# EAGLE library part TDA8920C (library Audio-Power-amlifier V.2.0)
The TDA8920C is a high-efficiency class-D audio power amplifier. The typical output power is 2 ´ 110 W with a speaker load impedance of 4 W. The TDA8920C is available in both HSOP24 and DBS23P power packages. The amplifier operates over a wide supply voltage range from ±12.5 V to ±32.5 V and features low quiescent current consumption.
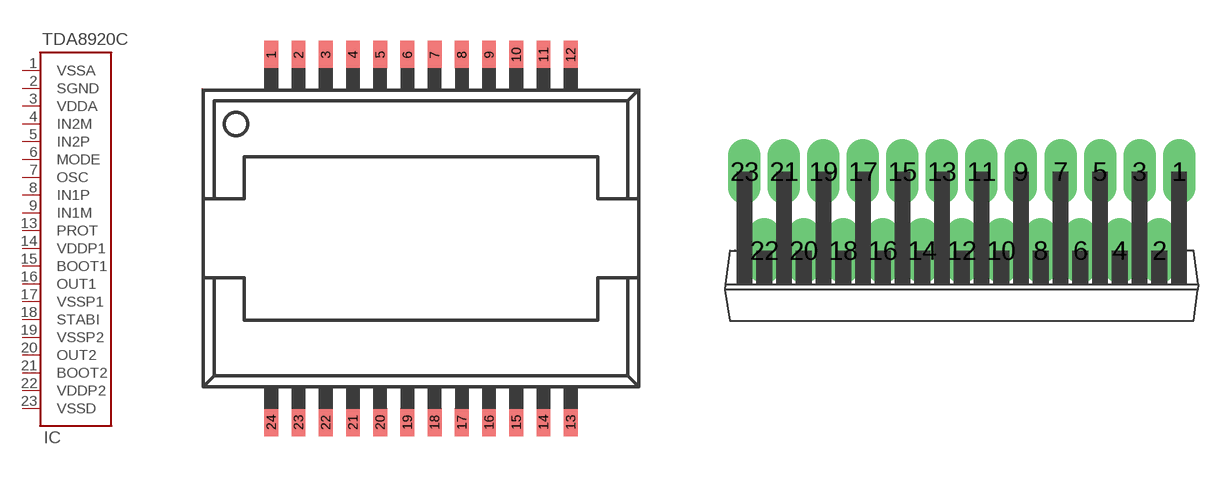
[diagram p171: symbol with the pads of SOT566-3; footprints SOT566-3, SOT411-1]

Designator prefix IC

## TDA8920CTDA8920CTH  [SOT566-3]
1  VSSA  pwr
2  SGND  pwr
3  VDDA  pwr
4  IN2M  in
5  IN2P  in
6  MODE  in
7  OSC  in
8  IN1P  in
9  IN1M  in
13  PROT
14  VDDP1  pwr
15  BOOT1
16  OUT1  out
17  VSSP1  pwr
18  STABI  pwr
19  VSSP2  pwr
20  OUT2
21  BOOT2  out
22  VDDP2  pwr
23  VSSD  pwr

## TDA8920CTDA8920CJ  [SOT411-1]
1  MODE  in
2  IN2P  in
3  IN2M  in
4  VDDA  pwr
5  SGND  pwr
6  VSSA  pwr
7  VSSD  pwr
8  VDDP2  pwr
9  BOOT2  out
10  OUT2
11  VSSP2  pwr
12  STABI  pwr
13  VSSP1  pwr
14  OUT1  out
15  BOOT1
16  VDDP1  pwr
17  PROT
21  IN1M  in
22  IN1P  in
23  OSC  in

## Footprint SOT566-3 (pad centres in mm)
smd 0.508 x 1.016: 1 -5.5,6.75; 2 -4.5,6.75; 3 -3.5,6.75; 4 -2.5,6.75; 5 -1.5,6.75; 6 -0.5,6.75; 7 0.5,6.75; 8 1.5,6.75; 9 2.5,6.75; 10 3.5,6.75; 11 4.5,6.75; 12 5.5,6.75; 13 5.5,-6.75; 14 4.5,-6.75; 15 3.5,-6.75; 16 2.5,-6.75; 17 1.5,-6.75; 18 0.5,-6.75; 19 -0.5,-6.75; 20 -1.5,-6.75; 21 -2.5,-6.75; 22 -3.5,-6.75; 23 -4.5,-6.75; 24 -5.5,-6.75

## Footprint SOT411-1 (pad centres in mm)
drill 1.4 long: 1 13.97,5.08; 2 12.7,0; 3 11.43,5.08; 4 10.16,0; 5 8.89,5.08; 6 7.62,0; 7 6.35,5.08; 8 5.08,0; 9 3.81,5.08; 10 2.54,0; 11 1.27,5.08; 12 0,0; 13 -1.27,5.08; 14 -2.54,0; 15 -3.81,5.08; 16 -5.08,0; 17 -6.35,5.08; 18 -7.62,0; 19 -8.89,5.08; 20 -10.16,0; 21 -11.43,5.08; 22 -12.7,0; 23 -13.97,5.08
